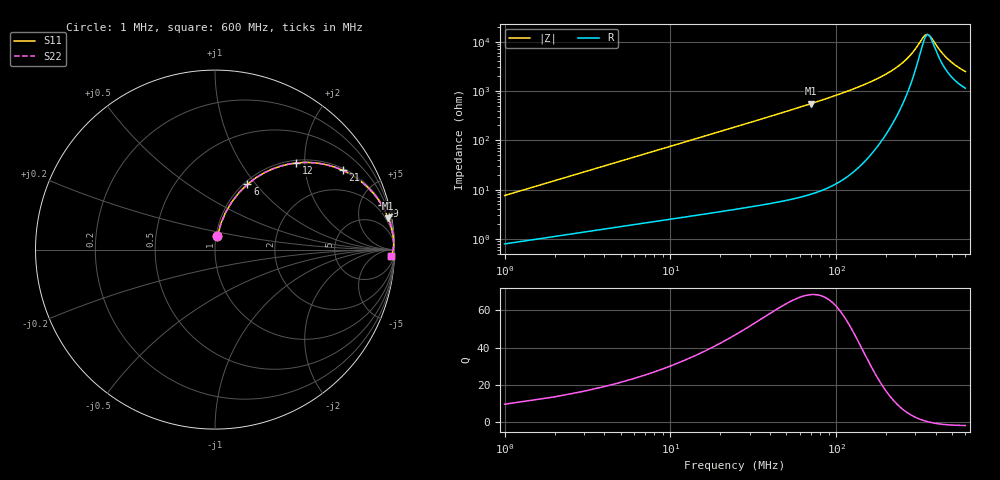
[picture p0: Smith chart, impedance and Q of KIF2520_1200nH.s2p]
!version-2
!date-12.2020
!Series
# MHz S RI R 50
!Freq ReS11 ImS11 ReS21 ImS21 ReS12 ImS12 ReS22 ImS22
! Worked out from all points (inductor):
!   600 points, 1 MHz to 600 MHz, reference 50 ohm
!   read as one part in series: L = 1.2 uH near 4 MHz
!   highest Q = 68.5 at 70 MHz (marker M1), where L = 1.25 uH
!   self-resonance near 358.8 MHz
!   S11 on the Smith chart (normalised r, x): 1 MHz: 1.02, +0.15; 6 MHz: 1.04, +0.91; 12 MHz: 1.05, +1.81; 21 MHz: 1.07, +3.18; 49 MHz: 1.12, +7.53; 600 MHz: 24, -44
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1  0.0134 0.0738  0.9866 -0.0738  0.9866 -0.0738  0.0134 0.0738
5  0.136 0.3201  0.864 -0.3201  0.864 -0.3201  0.136 0.3201
6  0.1805 0.3638  0.8195 -0.3638  0.8195 -0.3638  0.1805 0.3638
9  0.3216 0.4499  0.6784 -0.4499  0.6784 -0.4499  0.3216 0.4499
12  0.4524 0.4828  0.5476 -0.4828  0.5476 -0.4828  0.4524 0.4828
16  0.5915 0.4786  0.4085 -0.4786  0.4085 -0.4786  0.5915 0.4786
21  0.712 0.4415  0.288 -0.4415  0.288 -0.4415  0.712 0.4415
26  0.7905 0.3967  0.2095 -0.3967  0.2095 -0.3967  0.7905 0.3967
32  0.8509 0.3469  0.1491 -0.3469  0.1491 -0.3469  0.8509 0.3469
49  0.9308 0.246  0.0692 -0.246  0.0692 -0.246  0.9308 0.246
70  0.9655 0.1752  0.0345 -0.1752  0.0345 -0.1752  0.9655 0.1752
101  0.9838 0.1184  0.0162 -0.1184  0.0162 -0.1184  0.9838 0.1184
201  0.9953 0.0444  0.00474 -0.0444  0.00474 -0.0444  0.9953 0.0444
258  0.9954 0.0241  0.00463 -0.0241  0.00463 -0.0241  0.9954 0.0241
301  0.9946 0.0126  0.00544 -0.0126  0.00544 -0.0126  0.9946 0.0126
334  0.9936 0.00507  0.00638 -0.00507  0.00638 -0.00507  0.9936 0.00507
351  0.993 0.00154  0.00695 -0.00154  0.00695 -0.00154  0.993 0.00154
368  0.9924 -0.00178  0.00758 0.00178  0.00758 0.00178  0.9924 -0.00178
401  0.9911 -0.00774  0.00893 0.00774  0.00893 0.00774  0.9911 -0.00774
446  0.989 -0.015  0.011 0.015  0.011 0.015  0.989 -0.015
501  0.9862 -0.0228  0.0138 0.0228  0.0138 0.0228  0.9862 -0.0228
600  0.9804 -0.0347  0.0196 0.0347  0.0196 0.0347  0.9804 -0.0347
